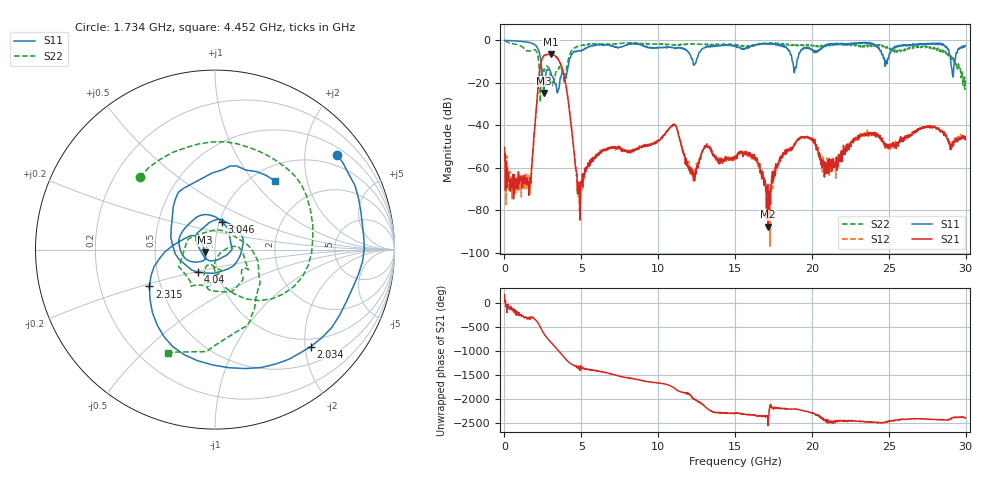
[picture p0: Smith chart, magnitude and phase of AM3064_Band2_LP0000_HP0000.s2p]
# Hz S DB R 50.0
!freq dBS11 angS11 dBS21 angS21 dBS12 angS12 dBS22 angS22
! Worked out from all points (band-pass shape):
!   1600 points, 10 MHz to 29.98 GHz, reference 50 ohm
!   highest |S21| = -6.50 dB at 3.028 GHz (marker M1); lowest = -87.6 dB at 17.14 GHz (marker M2)
!   |S21| within 3 dB of the highest: 2.409 GHz to 3.538 GHz (1.13 GHz wide, 38 % of centre)
!   lowest |S11| = -24.8 dB at 2.559 GHz (marker M3), VSWR 1.12, Z = 44.7 - j1.37 ohm
!   |S11| at or under -10 dB: 2.371 GHz to 4.2 GHz (1.829 GHz wide, 55.7 % of centre); 18.73 GHz to 19.02 GHz (288.3 MHz wide, 1.53 % of centre); 29.03 GHz to 29.26 GHz (230.3 MHz wide, 0.79 % of centre)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
!   |S22| runs from -29.0 to -0.2 dB; largest |S21 - S12| = 0.012
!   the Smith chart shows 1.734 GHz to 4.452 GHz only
!   S11 on the Smith chart (normalised r, x): 1.734 GHz: 0.67, +2.77; 2.034 GHz: 0.83, -2.12; 2.315 GHz: 0.43, -0.22; 3.046 GHz: 1.03, +0.33; 4.04 GHz: 0.81, -0.21; 4.452 GHz: 1.27, +1.30
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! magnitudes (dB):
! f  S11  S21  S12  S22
! 10 MHz  -0.1  -50.3  -57.5  -0.2
! 1.734 GHz  -1.3  -64.4  -61.7  -4.7
! 2.034 GHz  -2.4  -35.5  -35.4  -4.8
! 2.315 GHz  -7.6  -13.0  -12.9  -25.5
! 2.559 GHz  -24.8  -7.3  -7.3  -14.4
! 3.028 GHz  -15.5  -6.5  -6.5  -18.3
! 3.046 GHz  -16.0  -6.5  -6.5  -19.2
! 4.04 GHz  -16.1  -23.0  -22.9  -13.0
! 4.452 GHz  -5.9  -47.3  -47.5  -3.9
! 5.015 GHz  -4.9  -66.2  -68.7  -2.5
! 6.364 GHz  -2.1  -51.5  -52.2  -1.7
! 10 GHz  -3.4  -47.3  -47.0  -1.7
! 11.09 GHz  -3.8  -39.8  -39.7  -2.0
! 12.31 GHz  -11.6  -66.2  -64.7  -1.6
! 15 GHz  -2.6  -55.5  -56.2  -1.8
! 16.32 GHz  -2.1  -56.4  -54.7  -2.0
! 17.14 GHz  -1.6  -87.6  -83.3  -1.3
! 18.14 GHz  -3.1  -53.9  -53.8  -1.8
! 19.99 GHz  -4.3  -46.7  -46.7  -2.2
! 20.97 GHz  -2.5  -57.7  -57.1  -2.5
! 25 GHz  -8.1  -51.0  -50.2  -3.2
! 29.98 GHz  -2.5  -46.7  -46.8  -17.3
